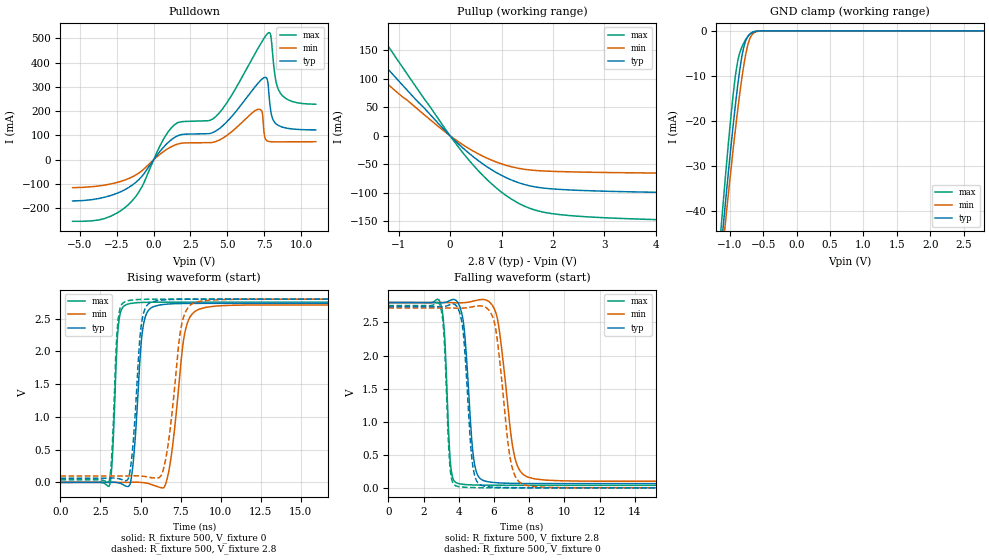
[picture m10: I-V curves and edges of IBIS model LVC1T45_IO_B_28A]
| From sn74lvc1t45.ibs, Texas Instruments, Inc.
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[Model]   LVC1T45_IO_B_28A
Model_type  I/O
Vinl=0.7
Vinh=1.7
Enable   Active-Low
Vref =   0
Rref =   2000
Cref =   15p
Vmeas =   1.25
| variable   typ   min   max
C_comp   7.03pF   6.20pF   8.18pF
| C_pullup   10.99pF   9.76pF   12.53pF
| C_pulldown   10.57pF   7.61pF   14.13pF
| C_tri-state   7.03pF   6.20pF   8.18pF
[Temperature Range]   40   100   -40
| Ambient temperature   25   85   -40
[Voltage range]   2.8   2.8   2.8
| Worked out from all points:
|   slope of the pulldown table from 0 to 0.42 V, typ, clamps not added: 12.3 ohm
|   slope of the pullup table from 0 to 0.42 V, typ, clamps not added: 12.2 ohm
|   GND clamp passes 1 mA (typ) near -0.71 V on its own axis
|   rising waveform, R_fixture 500, V_fixture 0: 20-80 % time 434ps typ, 689ps min, 276ps max; typ from 0 V to 2.74 V
|   falling waveform, R_fixture 500, V_fixture 2.8: 20-80 % time 417ps typ, 691ps min, 267ps max; typ from 2.8 V to 0.064 V
|   rising waveform, R_fixture 500, V_fixture 2.8: 20-80 % time 436ps typ, 703ps min, 278ps max; typ from 0.064 V to 2.8 V
|   falling waveform, R_fixture 500, V_fixture 0: 20-80 % time 402ps typ, 646ps min, 260ps max; typ from 2.74 V to 0 V
[GND Clamp]
| LVC1T45_IO_B_28A
|   Voltage   I(typ)   I(min)   I(max)
-5.5V     -910.9mA   -836.3mA   -1.031A
-1.14V    -50.34mA   -53.89mA   -45.85mA
-1.12V    -47.12mA   -50.9mA    -42.25mA
-1.075V   -39.97mA   -44.24mA   -34.35mA
-1.06V    -37.63mA   -42.05mA   -31.78mA
-960mV    -22.72mA   -27.97mA   -15.92mA
-880mV    -12.18mA   -17.61mA   -6.789mA
-825mV    -6.376mA   -11.28mA   -3.86mA
-775mV    -2.883mA   -6.453mA   -2.321mA
-710mV    -920.7uA   -2.212mA   -923.3uA
-645mV    -272.8uA   -519.5uA   -223.5uA
2.8V      8.953pA    15.32pA    7.945pA
[Pulldown]
| LVC1T45_IO_B_28A
|   Voltage   I(typ)   I(min)   I(max)
-5.5V     -169.9mA   -115.2mA   -253.7mA
-1.66V    -113.2mA   -76.45mA   -181.9mA
1.14V     79.49mA    51.82mA    127.3mA
4.225V    118.6mA    75.2mA     178.6mA
7.06V     313.9mA    207.7mA    457mA
7.365V    333.2mA    195.9mA    488.5mA
7.63V     338.4mA    81.63mA    512.9mA
7.805V    284.3mA    75.6mA     523.7mA
8.05V     173.3mA    73.9mA     453.3mA
8.28V     149.7mA    73.74mA    330mA
8.59V     137.7mA    73.76mA    275.3mA
11V       123mA      74.29mA    229mA
[Pullup]
| LVC1T45_IO_B_28A
|   Voltage   I(typ)   I(min)   I(max)
-5.5V     502.5mA    406.7mA    653.4mA
-2.51V    245.6mA    193.2mA    325.5mA
-2.015V   197.4mA    154.2mA    263mA
-1.895V   185.6mA    144.7mA    247.6mA
-1.435V   139.8mA    108.1mA    187.6mA
-20mV     1.83mA     1.366mA    2.531mA
460mV     -37.46mA   -27.37mA   -52.51mA
1.115V    -74.5mA    -52.48mA   -106.5mA
1.725V    -90.7mA    -61.27mA   -132.2mA
2.32V     -95.02mA   -63.26mA   -140mA
3.68V     -98.63mA   -65.12mA   -146.2mA
11V       -106.1mA   -69.35mA   -159mA
[Ramp]
| LVC1T45_IO_B_28A
| variable   typ   min   max
dV/dt_r   1.68/4.51E-10   1.68/7.19E-10   1.69/2.87E-10
dV/dt_f   1.67/4.32E-10   1.65/7.03E-10   1.69/2.77E-10
R_load = 500
[Rising Waveform]
| LVC1T45_IO_B_28A
R_fixture =   500
C_fixture =   0
L_fixture =   0
V_fixture =   0
V_fixture_min = 0
V_fixture_max = 0
|   Time   V(typ)   V(min)   V(max)
0s        154.7pV    326.9pV    90.5pV
3.05ns    1.159mV    18.75uV    -56.14mV
3.62ns    -6.99mV    -110uV     2.403V
4.19ns    -63.39mV   798.2uV    2.723V
5.12ns    2.311V     -2.132mV   2.75V
5.825ns   2.686V     -45.03mV   2.753V
6.655ns   2.724V     48.95mV    2.754V
7.755ns   2.734V     2.272V     2.754V
8.675ns   2.735V     2.648V     2.754V
34.99ns   2.736V     2.713V     2.754V
[Falling Waveform]
| LVC1T45_IO_B_28A
R_fixture =   500
C_fixture =   0
L_fixture =   0
V_fixture =   2.8
V_fixture_min = 2.8
V_fixture_max = 2.8
|   Time   V(typ)   V(min)   V(max)
0s        2.8V       2.8V       2.8V
2.94ns    2.797V     2.8V       2.807V
3.19ns    2.801V     2.8V       2.325V
3.54ns    2.836V     2.799V     339mV
3.955ns   2.798V     2.797V     67.93mV
4.865ns   413.9mV    2.825V     43.72mV
5.44ns    107.4mV    2.846V     40.79mV
7.195ns   67.75mV    450mV      38.76mV
7.985ns   65.61mV    157.2mV    38.59mV
34.99ns   63.86mV    97.93mV    38.4mV
[Rising Waveform]
| LVC1T45_IO_B_28A
R_fixture =   500
C_fixture =   0
L_fixture =   0
V_fixture =   2.8
V_fixture_min = 2.8
V_fixture_max = 2.8
|   Time   V(typ)   V(min)   V(max)
0s        63.77mV    97.78mV    38.36mV
3.045ns   64.86mV    97.8mV     18.41mV
3.575ns   59.04mV    97.68mV    2.425V
4.115ns   27.68mV    98.28mV    2.768V
5.06ns    2.423V     96.27mV    2.796V
5.7ns     2.757V     70.45mV    2.799V
6.47ns    2.788V     242.5mV    2.8V
7.52ns    2.798V     2.352V     2.8V
8.385ns   2.799V     2.748V     2.8V
34.99ns   2.8V       2.8V       2.8V
[Falling Waveform]
| LVC1T45_IO_B_28A
R_fixture =   500
C_fixture =   0
L_fixture =   0
V_fixture =   0
V_fixture_min = 0
V_fixture_max = 0
|   Time   V(typ)   V(min)   V(max)
0s        2.739V     2.718V     2.756V
2.925ns   2.736V     2.718V     2.761V
3.51ns    2.769V     2.718V     295.5mV
3.89ns    2.742V     2.716V     25.35mV
4.255ns   2.349V     2.717V     10.95mV
4.795ns   337.3mV    2.737V     4.365mV
5.325ns   35.08mV    2.747V     2.078mV
6.045ns   9.593mV    2.479V     886.1uV
7.72ns    1.333mV    45.35mV    223.1uV
34.99ns   77.34uV    133.9uV    39.5uV
